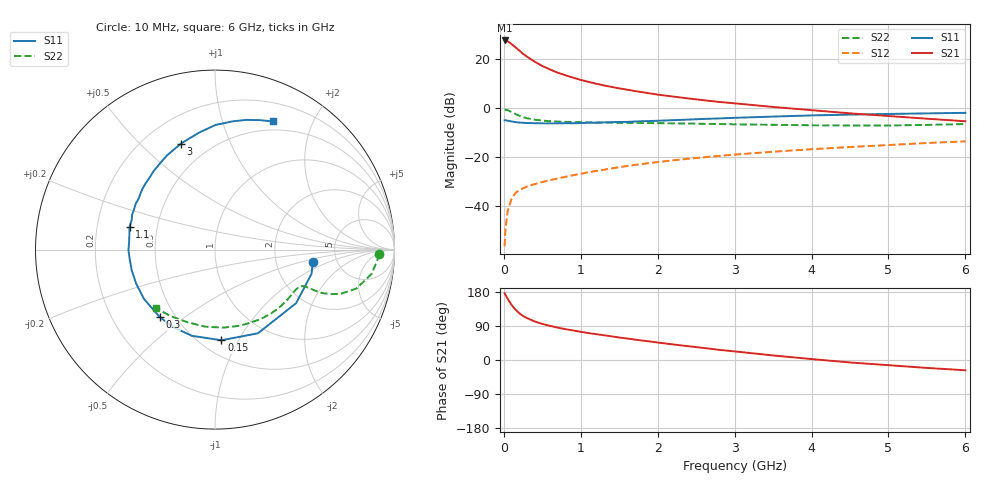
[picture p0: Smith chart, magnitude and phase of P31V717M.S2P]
! SIEMENS Small Signal Semiconductors
! BFP181
! Si NPN RF Bipolar Junction Transistor in SOT143
! VCE = 1.75 V  IC = 17 mA
! Common Emitter S-Parameters:  March  1996
# GHz  S  MA  R  50
!  f  S11  S21  S12  S22
! GHz  MAG  ANG  MAG  ANG  MAG  ANG  MAG  ANG
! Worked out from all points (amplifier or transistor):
!   36 points, 10 MHz to 6 GHz, reference 50 ohm
!   highest |S21| = 27.4 dB at 10 MHz (marker M1)
!   |S21| within 3 dB of that: start of sweep to 159.2 MHz
!   unconditionally stable (mu >= 1): start of sweep to 17.38 MHz; 397.1 MHz to end of sweep
!   at 250 MHz: K = 0.74, MSG = 27.4 dB, |S12| = -32.9 dB
!   at 1.4 GHz: K = 1.67, MAG = 11.8 dB, |S12| = -24.8 dB
!   at 6 GHz: K = 1.30, MAG = 0.8 dB, |S12| = -13.7 dB
!   S11 on the Smith chart (normalised r, x): 10 MHz: 3.31, -0.64; 150 MHz: 0.63, -0.85; 300 MHz: 0.41, -0.41; 1.1 GHz: 0.34, +0.12; 3 GHz: 0.35, +0.67; 6 GHz: 0.40, +1.47
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0.01  0.5497 -7.0  23.42 176.2  0.0015 73.8  0.9116 -1.5
0.02  0.5544 -14.1  23.33 172.7  0.0032 78.8  0.9076 -3.4
0.05  0.5417 -33.4  22.52 161.4  0.0078 78.3  0.8842 -8.7
0.1  0.5241 -62.9  19.78 145.6  0.0138 64.1  0.8173 -15.4
0.15  0.5063 -86.0  17.05 133.0  0.0181 57.2  0.7442 -19.3
0.2  0.4972 -105.0  14.64 123.6  0.0208 52.0  0.6864 -21.2
0.25  0.4908 -118.5  12.53 116.2  0.0227 49.6  0.6413 -22.1
0.3  0.4857 -129.4  10.98 110.7  0.0246 48.8  0.609 -22.3
0.4  0.4817 -145.3  8.666 101.8  0.0276 48.0  0.5683 -22.2
0.5  0.4785 -156.9  7.059 95.2  0.0305 48.1  0.5437 -22.3
0.6  0.4782 -166.1  6.002 90.0  0.0333 49.8  0.5292 -22.6
0.7  0.4781 -173.4  5.151 85.4  0.036 51.3  0.5191 -23.1
0.8  0.4822 -179.6  4.575 81.4  0.0389 52.2  0.5129 -23.9
1  0.4847 169.7  3.674 74.4  0.0446 53.4  0.5035 -26.0
1.1  0.4928 165.0  3.359 71.0  0.0484 53.8  0.5008 -27.2
1.5  0.5106 150.0  2.47 59.3  0.0612 54.8  0.4922 -32.8
2.2  0.5556 127.8  1.683 41.1  0.0842 52.7  0.4781 -44.7
3  0.6205 107.8  1.225 22.7  0.1104 47.6  0.4568 -60.6
3.5  0.6573 97.9  1.033 12.0  0.1262 44.1  0.4466 -71.8
4.5  0.7211 82.2  0.766 -6.5  0.1575 35.8  0.4327 -97.3
5.5  0.7636 70.8  0.595 -20.9  0.1901 27.8  0.4449 -123.1
6  0.7834 65.7  0.528 -27.1  0.2055 23.1  0.4637 -135.5
